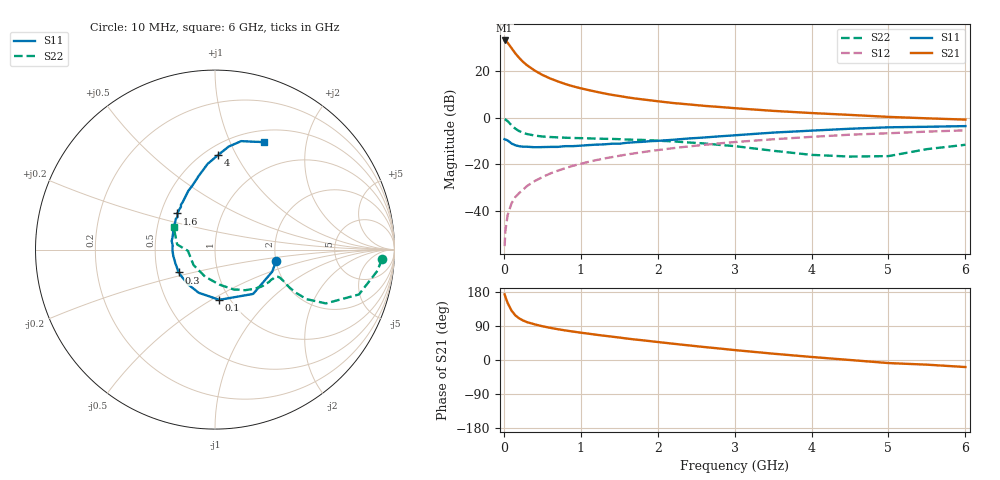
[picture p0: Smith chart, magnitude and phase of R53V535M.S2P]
! SIEMENS Small Signal Semiconductors
! BFR183
! Si NPN RF Bipolar Junction Transistor in SOT23
! VCE = 3.5 V  IC = 35 mA
! Common Emitter S-Parameters:  May  1996
# GHz  S  MA  R  50
!  f  S11  S21  S12  S22
! GHz  MAG  ANG  MAG  ANG  MAG  ANG  MAG  ANG
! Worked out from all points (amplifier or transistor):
!   36 points, 10 MHz to 6 GHz, reference 50 ohm
!   highest |S21| = 33.0 dB at 10 MHz (marker M1)
!   |S21| within 3 dB of that: start of sweep to 93.75 MHz
!   unconditionally stable (mu >= 1): 399.2 MHz to 2.336 GHz
!   at 250 MHz: K = 0.93, MSG = 27.3 dB, |S12| = -30.8 dB
!   at 1.4 GHz: K = 1.05, MAG = 12.0 dB, |S12| = -16.9 dB
!   at 6 GHz: K = 0.91, MSG = 2.3 dB, |S12| = -5.4 dB
!   S11 on the Smith chart (normalised r, x): 10 MHz: 2.01, -0.29; 100 MHz: 0.89, -0.54; 300 MHz: 0.64, -0.17; 1.6 GHz: 0.61, +0.27; 4 GHz: 0.58, +0.85; 6 GHz: 0.64, +1.36
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0.01  0.3463 -10.5  44.49 173.3  0.0018 82.6  0.9313 -3.3
0.02  0.3416 -21.2  44.02 166.8  0.0038 83.0  0.9129 -7.4
0.05  0.3258 -49.3  39.69 150.1  0.0084 78.9  0.8402 -17.3
0.1  0.2809 -85.1  30.47 130.3  0.0148 72.6  0.6865 -25.9
0.15  0.2571 -110.7  23.51 117.6  0.0202 71.1  0.5806 -28.4
0.2  0.2451 -126.6  18.84 109.8  0.0246 72.1  0.5155 -28.1
0.25  0.2395 -138.8  15.52 104.3  0.029 72.2  0.4731 -27.2
0.3  0.2393 -147.8  13.21 100.0  0.0345 73.9  0.4472 -26.2
0.4  0.2334 -161.8  10.15 94.1  0.0442 74.4  0.4148 -24.4
0.5  0.2351 -171.8  8.189 89.1  0.0535 74.6  0.3956 -23.5
0.6  0.2372 -179.2  6.886 85.0  0.0639 74.5  0.3862 -23.3
0.8  0.2461 168.8  5.216 78.0  0.0835 73.6  0.3726 -23.9
0.9  0.2463 163.9  4.661 75.0  0.0938 72.8  0.3677 -24.5
1.1  0.2593 154.2  3.878 69.5  0.1135 71.3  0.3609 -26.9
1.3  0.2684 145.9  3.303 64.2  0.1339 69.2  0.3533 -29.2
1.6  0.2909 136.1  2.721 56.6  0.1634 66.1  0.3408 -33.9
2.2  0.3368 119.4  2.053 43.0  0.2228 59.3  0.3112 -44.7
3.5  0.4793 94.9  1.396 16.7  0.3452 42.3  0.1962 -83.0
4  0.5277 88.1  1.254 8.0  0.3887 36.1  0.1604 -110.4
4.5  0.5793 82.4  1.144 0.0  0.4324 29.3  0.1474 -144.2
5.5  0.6383 70.3  0.967 -12.3  0.5032 17.3  0.2126 172.3
6  0.6595 65.3  0.908 -18.6  0.5359 9.7  0.2633 151.2
